| IBIS file stm32u595_599_5a5_5a9_tfbga216_dsi_smps.ibs
[IBIS ver] 4.2
[File name] stm32u595_599_5a5_5a9_tfbga216_dsi_smps.ibs
[File Rev] rev2.0
[Date]  11-09-2023
[Source] Data Created at STMicroelectronics
[Notes]  File originated from ELDO simulations.
[Disclaimer]  This information is for modeling purpose only and is
   not guaranteed. The information is subject to change without
   notice.
[Copyright] Copyright 2023 STMicroelectronics Inc.
|   Component stm32u595_599_5a5_5a9_tfbga216_dsi_smps
[Component] stm32u595_599_5a5_5a9_tfbga216_dsi_smps
[Manufacturer] STMicroelectronics
[Package]
| variable   typ   min   max
R_pkg  0  NA  NA
L_pkg  0  NA  NA
C_pkg  0  NA  NA
[Pin]   signal_name   model_name
A1  VSS  gnd
A2  PE0  io8_100m_hslv_ft
A3  PB7  io8_spi_hslv_ft
A4  PB6  io8_100m_i2c_ft
A5  PG15  io8_100m_hslv_ft
A6  PG12  io8_100m_hslv_ft
A7  PG9  io8_100m_hslv_ft
A8  PD4  io8_100m_hslv_ft
A9  PD3  io8_166m_hslv_ft
A10  PC10  io8_100m_ft
A11  PA15  nc
A12  PA14  io8_100m_ft
A13  PA8  io8_166m_hslv_ft
A14  PC8  io8_100m_ft
A15  VSS  gnd
B1  PC14-OSC32_IN  nc
B2  PE4  io8_100m_hslv_tamp_ft
B3  PE1  io8_100m_hslv_ft
B4  PH3-BOOT0  nc
B5  PB5  io8_166m_hslv_ft
B6  PG13  io8_100m_hslv_ft
B7  PG10  io8_100m_hslv_ft
B8  PD5  io8_100m_hslv_ft
B9  PD2  io8_100m_ft
B10  PC11  io8_100m_hslv_ft
B11  PH7  io8_spi_hslv_ft
B12  PH5  io8_100m_i2c_ft
B13  PA12  io8_100m_ft
B14  PA11  io8_100m_ft
B15  PC7  io8_100m_ft
C1  PC15-OSC32_OUT  nc
C2  VBAT  power
C3  PE3  io8_100m_hslv_tamp_ft
C4  PI5  io8_100m_hslv_ft
C5  PB9  io8_100m_i2c_ft
C6  PB8  io8_100m_i2c_ft
C7  PG11  io8_100m_hslv_ft
C8  PD6  io8_166m_hslv_ft
C9  PD1  io8_100m_hslv_ft
C10  PC12  io8_166m_hslv_ft
C11  PH6  io8_166m_hslv_ft
C12  PH4  io8_100m_hslv_ft
C13  PA13  io8_100m_ft
C14  PC9  io8_100m_ft
C15  PC6  io8_100m_ft
D1  PJ3  io8_100m_ft
D2  PJ2  io8_100m_ft
D3  PE5  io8_100m_hslv_tamp_ft
D4  PI7  io8_spi_ft
D5  PI6  io8_spi_ft
D6  PB4  io8_100m_i2c_ft
D7  PG14  io8_100m_hslv_ft
D8  PD7  io8_100m_hslv_ft
D9  PD0  io8_100m_hslv_ft
D10  PH8  io8_100m_hslv_ft
D11  PH2  io8_100m_hslv_ft
D12  PA10  io8_100m_usb_id
D13  PG7  io8_100m_hslv_ft
D14  PG6  io8_100m_hslv_ft
D15  PG3  io8_100m_hslv_ft
E1  PJ7  io8_100m_ft
E2  PJ6  io8_100m_ft
E3  PJ4  io8_100m_ft
E4  PE6  io8_100m_hslv_tamp_ft
E5  PE2  io8_100m_hslv_ft
E6  VDD11  nc
E7  PB3  io8_100m_i2c_ft
E8  VDDIO2  power
E9  VDDUSB  power
E10  VSS  gnd
E11  VDD11  nc
E12  PA9  io8_100m_usb_vbus_ft
E13  PG8  io8_100m_i2c_ft
E14  PG5  io8_100m_hslv_ft
E15  PJ0  io8_spi_ft
F1  PJ10  io8_100m_ft
F2  PJ8  io8_100m_ft
F3  PJ5  io8_100m_ft
F4  PC13  io8_100m_ft
F5  VDD  power
F6  VSS  gnd
F7  VSS  gnd
F8  VDD  power
F9  VSS  gnd
F10  VSS  gnd
F11  VDD11USB  nc
F12  PG4  io8_100m_hslv_ft
F13  PI15  io8_spi_ft
F14  PI14  io8_spi_ft
F15  PI13  io8_spi_ft
G1  DSI_D0P  nc
G2  DSI_D0N  nc
G3  PJ11  io8_100m_ft
G4  PJ1  io8_100m_ft
G5  VDDDSI  nc
G6  VSSDSI  nc
G10  VSS  gnd
G11  VDDIO2  power
G12  PG2  io8_100m_hslv_ft
G13  PI12  io8_spi_ft
G14  PI11  io8_spi_ft
G15  PI10  io8_spi_ft
H1  DSI_CKP  nc
H2  VSSDSI  nc
H3  PF0  io8_100m_hslv_ft
H4  PJ9  io8_100m_ft
H5  VDD11DSI  nc
H6  VSSDSI  nc
H10  VSS  gnd
H11  VDD  power
H12  PI9  io8_spi_ft
H13  PI8  io8_spi_ft
H14  PI4  io8_spi_ft
H15  VSS  gnd
J1  DSI_CKN  nc
J2  VSSDSI  nc
J3  PF2  io8_100m_hslv_ft
J4  PF1  io8_100m_hslv_ft
J5  VDD  power
J6  VSS  gnd
J10  VSS  gnd
J11  VDD_HSPI  power
J12  PI1  io8_spi_ft
J13  PI2  io8_spi_ft
J14  PI3  io8_spi_ft
J15  VSS  gnd
K1  DSI_D1N  nc
K2  DSI_D1P  nc
K3  PF4  io8_spi_ft
K4  PF3  io8_100m_hslv_ft
K5  VREFM  nc
K6  VSSA  nc
K7  VSS  gnd
K8  VSS  gnd
K9  VSS  gnd
K10  VSS  gnd
K11  VDD  power
K12  PD15  io8_100m_hslv_ft
K13  PH14  io8_spi_ft
K14  PH15  io8_spi_ft
K15  PI0  io8_spi_ft
L1  PF10  io8_166m_hslv_ft
L2  PF5  io8_spi_ft
L3  PF7  io8_100m_hslv_ft
L4  PF9  io8_100m_hslv_ft
L5  VREFP  nc
L6  VDDA  nc
L7  VDD  power
L8  VDD  power
L9  VDD  power
L10  VSS  gnd
L11  VDD power
L12  PD11  io8_100m_hslv_ft
L13  PH10  io8_spi_ft
L14  PH11  io8_spi_ft
L15  PH13  io8_spi_ft
M1  PC1  io8_spi_hslv_ft
M2  PF6  io8_100m_hslv_ft
M3  PF8  io8_100m_hslv_ft
M4  PA2  io8_100m_hslv_ft
M5  PA4  io8_100m_hslv_ft
M6  PB1  io8_100m_hslv_ft
M7  PF13  io8_100m_hslv_ft
M8  PE8  io8_100m_hslv_ft
M9  PE13  io8_100m_hslv_ft
M10  PB11  io8_100m_hslv_ft
M11  PB12  io8_166m_hslv_ft
M12  PB13  io8_100m_i2c_ft
M13  PD12  io8_100m_hslv_ft
M14  PH9  io8_spi_ft
M15  PH12  io8_spi_ft
N1  PH0-OSC_IN  nc
N2  PH1-OSC_OUT  nc
N3  PC3  io8_100m_hslv_ft
N4  PA0  io8_100m_hslv_tamp_ft
N5  OPAMP2_VINM  nc
N6  PB0  io8_100m_hslv_ft
N7  PF12  io8_100m_hslv_ft
N8  PG1  io8_100m_hslv_ft
N9  PE7  io8_100m_hslv_ft
N10  PE15  io8_100m_hslv_ft
N11  PE12  io8_100m_hslv_ft
N12  PB10  io8_spi_hslv_ft
N13  PD8  io8_100m_hslv_ft
N14  PD13  io8_100m_hslv_ft
N15  PD14  io8_100m_hslv_ft
P1  PC2  io8_100m_hslv_ft
P2  PC0  io8_100m_hslv_ft
P3  PA1  io8_100m_hslv_tamp_ft
P4  PA3  io8_166m_hslv_ft
P5  PA6  io8_100m_hslv_ft
P6  PC5  io8_100m_tamp_ft
P7  PF11  io8_166m_hslv_ft
P8  PF15  io8_100m_hslv_ft
P9  PE9  io8_166m_hslv_ft
P10  PE10  io8_166m_hslv_ft
P11  PE11  io8_100m_hslv_ft
P12  VSSSMPS  nc
P13  PB14  io8_100m_i2c_ft
P14  PD10  io8_100m_hslv_ft
P15  PD9  io8_100m_hslv_ft
R1  VSS  gnd
R2  NRST  nc
R3  OPAMP1_VINM  nc
R4  PA5  io8_100m_ft
R5  PA7  io8_100m_hslv_ft
R6  PC4  io8_100m_hslv_ft
R7  PB2  io8_100m_hslv_tamp_ft
R8  PF14  io8_100m_hslv_ft
R9  PG0  io8_100m_hslv_ft
R10  PE14  io8_100m_hslv_ft
R11  VLXSMPS  nc
R12  VDDSMPS  nc
R13  VDD11  nc
R14  PB15  nc
R15  VSS  gnd
[Package Model]   481-tfbga-13x13-216-220909
[Pin Mapping]   pulldown_ref   pullup_ref   | Comment
A1  gndio  nc
A2  gndio  vddiom
A3  gndio  vddiom
A4  gndio  vddiom
A5  gndio  vddiom  | Depending on IO usage
| A5  gndio  vddio2  | Depending on IO usage
A6  gndio  vddiom  | Depending on IO usage
| A6  gndio  vddio2  | Depending on IO usage
A7  gndio  vddiom  | Depending on IO usage
| A7  gndio  vddio2  | Depending on IO usage
A8  gndio  vddiom
A9  gndio  vddiom
A10  gndio  vddiom
A11  nc  nc
A12  gndio  vddiom
A13  gndio  vddiom
A14  gndio  vddiom
A15  gndio  nc
B1  nc  nc
B2  gndio  vddiom
B3  gndio  vddiom
B4  nc  nc
B5  gndio  vddiom
B6  gndio  vddiom  | Depending on IO usage
| B6  gndio  vddio2  | Depending on IO usage
B7  gndio  vddiom  | Depending on IO usage
| B7  gndio  vddio2  | Depending on IO usage
B8  gndio  vddiom
B9  gndio  vddiom
B10  gndio  vddiom
B11  gndio  vddiom
B12  gndio  vddiom
B13  gndio  vddiom  | Depending on IO usage
| B13  gndio  vddusb  | Depending on IO usage
B14  gndio  vddiom  | Depending on IO usage
| B14  gndio  vddusb  | Depending on IO usage
B15  gndio  vddiom
C1  nc  nc
C2  nc  vsw
C3  gndio  vddiom
C4  gndio  vddiom
C5  gndio  vddiom
C6  gndio  vddiom
C7  gndio  vddiom  | Depending on IO usage
| C7  gndio  vddio2  | Depending on IO usage
C8  gndio  vddiom
C9  gndio  vddiom
C10  gndio  vddiom
C11  gndio  vddiom
C12  gndio  vddiom
C13  gndio  vddiom  | Depending on IO usage
| C13  gndio  vddusb  | Depending on IO usage
C14  gndio  vddiom
C15  gndio  vddiom
D1  gndio  vddiom
D2  gndio  vddiom
D3  gndio  vddiom
D4  gndio  vddiom
D5  gndio  vddiom
D6  gndio  vddiom
D7  gndio  vddiom  | Depending on IO usage
| D7  gndio  vddio2  | Depending on IO usage
D8  gndio  vddiom
D9  gndio  vddiom
D10  gndio  vddiom
D11  gndio  vddiom
D12  gndio  vddiom  | Depending on IO usage
| D12  gndio  vddusb  | Depending on IO usage
D13  gndio  vddiom  | Depending on IO usage
| D13  gndio  vddio2  | Depending on IO usage
D14  gndio  vddiom  | Depending on IO usage
| D14  gndio  vddio2  | Depending on IO usage
D15  gndio  vddiom  | Depending on IO usage
| D15  gndio  vddio2  | Depending on IO usage
E1  gndio  vddiom
E2  gndio  vddiom
E3  gndio  vddiom
E4  gndio  vddiom
E5  gndio  vddiom
E6  nc  nc
E7  gndio  vddiom
E8  nc  vddio2
E9  nc  vddusb
E10  gndio  nc
E11  nc  nc
E12  gndio  vddiom  | Depending on IO usage
| E12  gndio  vddusb  | Depending on IO usage
E13  gndio  vddiom  | Depending on IO usage
| E13  gndio  vddio2  | Depending on IO usage
E14  gndio  vddiom  | Depending on IO usage
| E14  gndio  vddio2  | Depending on IO usage
E15  gndio  vddiom
F1  gndio  vddiom
F2  gndio  vddiom
F3  gndio  vddiom
F4  gndio  vddiom  | Depending on IO usage
| F4  gndio  vsw  | Depending on IO usage
F5  nc  vddiom
F6  gndio  nc
F7  gndio  nc
F8  nc  vddiom
F9  gndio  nc
F10  gndio  nc
F11  nc  nc
F12  gndio  vddiom  | Depending on IO usage
| F12  gndio  vddio2  | Depending on IO usage
F13  gndio  vddiom
F14  gndio  vddiom
F15  gndio  vddiom
G1  nc  nc
G2  nc  nc
G3  gndio  vddiom
G4  gndio  vddiom
G5  nc  nc
G6  nc  nc
G10  gndio  nc
G11  nc  vddio2
G12  gndio  vddiom  | Depending on IO usage
| G12  gndio  vddio2  | Depending on IO usage
G13  gndio  vddiom
G14  gndio  vddiom
G15  gndio  vddiom
H1  nc  nc
H2  nc  nc
H3  gndio  vddiom
H4  gndio  vddiom
H5  nc  nc
H6  nc  nc
H10  gndio  nc
H11  nc  vddhspi
H12  gndio  vddiom
H13  gndio  vddiom
H14  gndio  vddiom
H15  gndio  nc
J1  nc  nc
J2  nc  nc
J3  gndio  vddiom
J4  gndio  vddiom
J5  nc  vddiom
J6  gndio  nc
J10  gndio  nc
J11  nc  vddhspi
J12  gndio  vddiom
J13  gndio  vddiom
J14  gndio  vddiom
J15  gndio  nc
K1  nc  nc
K2  nc  nc
K3  gndio  vddiom
K4  gndio  vddiom
K5  nc  nc
K6  nc  nc
K7  gndio  nc
K8  gndio  nc
K9  gndio  nc
K10  gndio  nc
K11  nc  vddhspi
K12  gndio  vddiom
K13  gndio  vddiom
K14  gndio  vddiom
K15  gndio  vddiom
L1  gndio  vddiom
L2  gndio  vddiom
L3  gndio  vddiom
L4  gndio  vddiom
L5  nc  nc
L6  nc  nc
L7  nc  vddiom
L8  nc  vddiom
L9  nc  vddiom
L10  gndio  nc
L11  nc  vddhspi
L12  gndio  vddiom
L13  gndio  vddiom
L14  gndio  vddiom
L15  gndio  vddiom
M1  gndio  vddiom
M2  gndio  vddiom
M3  gndio  vddiom
M4  gndio  vddiom
M5  gndio  vddiom
M6  gndio  vddiom
M7  gndio  vddiom
M8  gndio  vddiom
M9  gndio  vddiom
M10  gndio  vddiom
M11  gndio  vddiom
M12  gndio  vddiom
M13  gndio  vddiom
M14  gndio  vddiom
M15  gndio  vddiom
N1  nc  nc
N2  nc  nc
N3  gndio  vddiom
N4  gndio  vddiom
N5  nc  nc
N6  gndio  vddiom
N7  gndio  vddiom
N8  gndio  vddiom
N9  gndio  vddiom
N10  gndio  vddiom
N11  gndio  vddiom
N12  gndio  vddiom
N13  gndio  vddiom
N14  gndio  vddiom
N15  gndio  vddiom
P1  gndio  vddiom
P2  gndio  vddiom
P3  gndio  vddiom
P4  gndio  vddiom
P5  gndio  vddiom
P6  gndio  vddiom
P7  gndio  vddiom
P8  gndio  vddiom
P9  gndio  vddiom
P10  gndio  vddiom
P11  gndio  vddiom
P12  nc  nc
P13  gndio  vddiom
P14  gndio  vddiom
P15  gndio  vddiom
R1  gndio  nc
R2  nc  nc
R3  nc  nc
R4  gndio  vddiom
R5  gndio  vddiom
R6  gndio  vddiom
R7  gndio  vddiom
R8  gndio  vddiom
R9  gndio  vddiom
R10  gndio  vddiom
R11  nc  nc
R12  nc  nc
R13  nc  nc
R14  nc  nc
R15  gndio  nc
[Model Selector] io8_100m_ft
io8_100m_ft_hs_1v2  "IO8_FT 100MHz high speed @ 1.2V"
io8_100m_ft_fs_1v2  "IO8_FT 100MHz fast speed @ 1.2V"
io8_100m_ft_fs_pd_1v2  "IO8_FT 100MHz fast speed @ 1.2V pulldown"
io8_100m_ft_ms_1v2  "IO8_FT 100MHz med speed @ 1.2V"
io8_100m_ft_ms_pd_1v2  "IO8_FT 100MHz med speed @ 1.2V pulldown"
io8_100m_ft_ls_1v2  "IO8_FT 100MHz low speed @ 1.2V"
io8_100m_ft_ls_pd_1v2  "IO8_FT 100MHz low speed @ 1.2V pulldown"
io8_100m_ft_hs_1v8  "IO8_FT 100MHz high speed @ 1.8V"
io8_100m_ft_hs_pd_1v8  "IO8_FT 100MHz high speed @ 1.8V pulldown"
io8_100m_ft_fs_1v8  "IO8_FT 100MHz fast speed @ 1.8V"
io8_100m_ft_fs_pd_1v8  "IO8_FT 100MHz fast speed @ 1.8V pulldown"
io8_100m_ft_ms_1v8  "IO8_FT 100MHz med speed @ 1.8V"
io8_100m_ft_ms_pd_1v8  "IO8_FT 100MHz med speed @ 1.8V pulldown"
io8_100m_ft_ls_1v8  "IO8_FT 100MHz low speed @ 1.8V"
io8_100m_ft_ls_pd_1v8  "IO8_FT 100MHz low speed @ 1.8V pulldown"
io8_100m_ft_hs_3v3  "IO8_FT 100MHz high speed @ 3.3V"
io8_100m_ft_hs_pd_3v3  "IO8_FT 100MHz high speed @ 3.3V pulldown"
io8_100m_ft_fs_3v3  "IO8_FT 100MHz fast speed @ 3.3V"
io8_100m_ft_fs_pd_3v3  "IO8_FT 100MHz fast speed @ 3.3V pulldown"
io8_100m_ft_ms_3v3  "IO8_FT 100MHz med speed @ 3.3V"
io8_100m_ft_ms_pd_3v3  "IO8_FT 100MHz med speed @ 3.3V pulldown"
io8_100m_ft_ls_3v3  "IO8_FT 100MHz low speed @ 3.3V"
io8_100m_ft_ls_pd_3v3  "IO8_FT 100MHz low speed @ 3.3V pulldown"
[Model Selector] io8_100m_hslv_ft
io8_100m_ft_hs_1v2  "IO8_FT 100MHz high speed @ 1.2V"
io8_100m_ft_hs_pu_1v2  "IO8_FT 100MHz high speed @ 1.2V pullup"
io8_100m_ft_hs_pd_1v2  "IO8_FT 100MHz high speed @ 1.2V pulldown"
io8_100m_ft_fs_1v2  "IO8_FT 100MHz fast speed @ 1.2V"
io8_100m_ft_fs_pu_1v2  "IO8_FT 100MHz fast speed @ 1.2V pullup"
io8_100m_ft_fs_pd_1v2  "IO8_FT 100MHz fast speed @ 1.2V pulldown"
io8_100m_ft_ms_1v2  "IO8_FT 100MHz med speed @ 1.2V"
io8_100m_ft_ms_pu_1v2  "IO8_FT 100MHz med speed @ 1.2V pullup"
io8_100m_ft_ms_pd_1v2  "IO8_FT 100MHz med speed @ 1.2V pulldown"
io8_100m_ft_ls_1v2  "IO8_FT 100MHz low speed @ 1.2V"
io8_100m_ft_ls_pu_1v2  "IO8_FT 100MHz low speed @ 1.2V pullup"
io8_100m_ft_ls_pd_1v2  "IO8_FT 100MHz low speed @ 1.2V pulldown"
io8_100m_ft_hs_1v8  "IO8_FT 100MHz high speed @ 1.8V"
io8_100m_ft_hs_pu_1v8  "IO8_FT 100MHz high speed @ 1.8V pullup"
io8_100m_ft_hs_pd_1v8  "IO8_FT 100MHz high speed @ 1.8V pulldown"
io8_100m_ft_fs_1v8  "IO8_FT 100MHz fast speed @ 1.8V"
io8_100m_ft_fs_pu_1v8  "IO8_FT 100MHz fast speed @ 1.8V pullup"
io8_100m_ft_fs_pd_1v8  "IO8_FT 100MHz fast speed @ 1.8V pulldown"
io8_100m_ft_ms_1v8  "IO8_FT 100MHz med speed @ 1.8V"
io8_100m_ft_ms_pu_1v8  "IO8_FT 100MHz med speed @ 1.8V pullup"
io8_100m_ft_ms_pd_1v8  "IO8_FT 100MHz med speed @ 1.8V pulldown"
io8_100m_ft_ls_1v8  "IO8_FT 100MHz low speed @ 1.8V"
io8_100m_ft_ls_pu_1v8  "IO8_FT 100MHz low speed @ 1.8V pullup"
io8_100m_ft_ls_pd_1v8  "IO8_FT 100MHz low speed @ 1.8V pulldown"
io8_100m_ft_hs_3v3  "IO8_FT 100MHz high speed @ 3.3V"
io8_100m_ft_hs_pu_3v3  "IO8_FT 100MHz high speed @ 3.3V pullup"
io8_100m_ft_hs_pd_3v3  "IO8_FT 100MHz high speed @ 3.3V pulldown"
io8_100m_ft_fs_3v3  "IO8_FT 100MHz fast speed @ 3.3V"
io8_100m_ft_fs_pu_3v3  "IO8_FT 100MHz fast speed @ 3.3V pullup"
io8_100m_ft_fs_pd_3v3  "IO8_FT 100MHz fast speed @ 3.3V pulldown"
io8_100m_ft_ms_3v3  "IO8_FT 100MHz med speed @ 3.3V"
io8_100m_ft_ms_pu_3v3  "IO8_FT 100MHz med speed @ 3.3V pullup"
io8_100m_ft_ms_pd_3v3  "IO8_FT 100MHz med speed @ 3.3V pulldown"
io8_100m_ft_ls_3v3  "IO8_FT 100MHz low speed @ 3.3V"
io8_100m_ft_ls_pu_3v3  "IO8_FT 100MHz low speed @ 3.3V pullup"
io8_100m_ft_ls_pd_3v3  "IO8_FT 100MHz low speed @ 3.3V pulldown"
io8_100m_hslv_ft_hs_1v2  "IO8_FT 100MHz HSLV high speed @ 1.2V"
io8_100m_hslv_ft_hs_pu_1v2  "IO8_FT 100MHz HSLV high speed @ 1.2V pullup"
io8_100m_hslv_ft_hs_pd_1v2  "IO8_FT 100MHz HSLV high speed @ 1.2V pulldown"
io8_100m_hslv_ft_fs_1v2  "IO8_FT 100MHz HSLV fast speed @ 1.2V"
io8_100m_hslv_ft_fs_pu_1v2  "IO8_FT 100MHz HSLV fast speed @ 1.2V pullup"
io8_100m_hslv_ft_fs_pd_1v2  "IO8_FT 100MHz HSLV fast speed @ 1.2V pulldown"
io8_100m_hslv_ft_ms_1v2  "IO8_FT 100MHz HSLV med speed @ 1.2V"
io8_100m_hslv_ft_ms_pu_1v2  "IO8_FT 100MHz HSLV med speed @ 1.2V pullup"
io8_100m_hslv_ft_ms_pd_1v2  "IO8_FT 100MHz HSLV med speed @ 1.2V pulldown"
io8_100m_hslv_ft_ls_1v2  "IO8_FT 100MHz HSLV low speed @ 1.2V"
io8_100m_hslv_ft_ls_pu_1v2  "IO8_FT 100MHz HSLV low speed @ 1.2V pullup"
io8_100m_hslv_ft_ls_pd_1v2  "IO8_FT 100MHz HSLV low speed @ 1.2V pulldown"
io8_100m_hslv_ft_hs_1v8  "IO8_FT 100MHz HSLV high speed @ 1.8V"
io8_100m_hslv_ft_hs_pu_1v8  "IO8_FT 100MHz HSLV high speed @ 1.8V pullup"
io8_100m_hslv_ft_hs_pd_1v8  "IO8_FT 100MHz HSLV high speed @ 1.8V pulldown"
io8_100m_hslv_ft_fs_1v8  "IO8_FT 100MHz HSLV fast speed @ 1.8V"
io8_100m_hslv_ft_fs_pu_1v8  "IO8_FT 100MHz HSLV fast speed @ 1.8V pullup"
io8_100m_hslv_ft_fs_pd_1v8  "IO8_FT 100MHz HSLV fast speed @ 1.8V pulldown"
io8_100m_hslv_ft_ms_1v8  "IO8_FT 100MHz HSLV med speed @ 1.8V"
io8_100m_hslv_ft_ms_pu_1v8  "IO8_FT 100MHz HSLV med speed @ 1.8V pullup"
io8_100m_hslv_ft_ms_pd_1v8  "IO8_FT 100MHz HSLV med speed @ 1.8V pulldown"
io8_100m_hslv_ft_ls_1v8  "IO8_FT 100MHz HSLV low speed @ 1.8V"
io8_100m_hslv_ft_ls_pu_1v8  "IO8_FT 100MHz HSLV low speed @ 1.8V pullup"
io8_100m_hslv_ft_ls_pd_1v8  "IO8_FT 100MHz HSLV low speed @ 1.8V pulldown"
io8_100m_hslv_ft_hs_2v5  "IO8_FT 100MHz HSLV high speed @ 2.5V"
io8_100m_hslv_ft_hs_pu_2v5  "IO8_FT 100MHz HSLV high speed @ 2.5V pullup"
io8_100m_hslv_ft_hs_pd_2v5  "IO8_FT 100MHz HSLV high speed @ 2.5V pulldown"
io8_100m_hslv_ft_fs_2v5  "IO8_FT 100MHz HSLV fast speed @ 2.5V"
io8_100m_hslv_ft_fs_pu_2v5  "IO8_FT 100MHz HSLV fast speed @ 2.5V pullup"
io8_100m_hslv_ft_fs_pd_2v5  "IO8_FT 100MHz HSLV fast speed @ 2.5V pulldown"
io8_100m_hslv_ft_ms_2v5  "IO8_FT 100MHz HSLV med speed @ 2.5V"
io8_100m_hslv_ft_ms_pu_2v5  "IO8_FT 100MHz HSLV med speed @ 2.5V pullup"
io8_100m_hslv_ft_ms_pd_2v5  "IO8_FT 100MHz HSLV med speed @ 2.5V pulldown"
io8_100m_hslv_ft_ls_2v5  "IO8_FT 100MHz HSLV low speed @ 2.5V"
io8_100m_hslv_ft_ls_pu_2v5  "IO8_FT 100MHz HSLV low speed @ 2.5V pullup"
io8_100m_hslv_ft_ls_pd_2v5  "IO8_FT 100MHz HSLV low speed @ 2.5V pulldown"
[Model Selector] io8_100m_hslv_tamp_ft
io8_100m_ft_hs_1v2  "IO8_FT 100MHz high speed @ 1.2V"
io8_100m_ft_hs_pu_1v2  "IO8_FT 100MHz high speed @ 1.2V pullup"
io8_100m_ft_hs_pd_1v2  "IO8_FT 100MHz high speed @ 1.2V pulldown"
io8_100m_ft_fs_1v2  "IO8_FT 100MHz fast speed @ 1.2V"
io8_100m_ft_fs_pu_1v2  "IO8_FT 100MHz fast speed @ 1.2V pullup"
io8_100m_ft_fs_pd_1v2  "IO8_FT 100MHz fast speed @ 1.2V pulldown"
io8_100m_ft_ms_1v2  "IO8_FT 100MHz med speed @ 1.2V"
io8_100m_ft_ms_pu_1v2  "IO8_FT 100MHz med speed @ 1.2V pullup"
io8_100m_ft_ms_pd_1v2  "IO8_FT 100MHz med speed @ 1.2V pulldown"
io8_100m_ft_ls_1v2  "IO8_FT 100MHz low speed @ 1.2V"
io8_100m_ft_ls_pu_1v2  "IO8_FT 100MHz low speed @ 1.2V pullup"
io8_100m_ft_ls_pd_1v2  "IO8_FT 100MHz low speed @ 1.2V pulldown"
io8_100m_ft_hs_1v8  "IO8_FT 100MHz high speed @ 1.8V"
io8_100m_ft_hs_pu_1v8  "IO8_FT 100MHz high speed @ 1.8V pullup"
io8_100m_ft_hs_pd_1v8  "IO8_FT 100MHz high speed @ 1.8V pulldown"
io8_100m_ft_fs_1v8  "IO8_FT 100MHz fast speed @ 1.8V"
io8_100m_ft_fs_pu_1v8  "IO8_FT 100MHz fast speed @ 1.8V pullup"
io8_100m_ft_fs_pd_1v8  "IO8_FT 100MHz fast speed @ 1.8V pulldown"
io8_100m_ft_ms_1v8  "IO8_FT 100MHz med speed @ 1.8V"
io8_100m_ft_ms_pu_1v8  "IO8_FT 100MHz med speed @ 1.8V pullup"
io8_100m_ft_ms_pd_1v8  "IO8_FT 100MHz med speed @ 1.8V pulldown"
io8_100m_ft_ls_1v8  "IO8_FT 100MHz low speed @ 1.8V"
io8_100m_ft_ls_pu_1v8  "IO8_FT 100MHz low speed @ 1.8V pullup"
io8_100m_ft_ls_pd_1v8  "IO8_FT 100MHz low speed @ 1.8V pulldown"
io8_100m_ft_hs_3v3  "IO8_FT 100MHz high speed @ 3.3V"
io8_100m_ft_hs_pu_3v3  "IO8_FT 100MHz high speed @ 3.3V pullup"
io8_100m_ft_hs_pd_3v3  "IO8_FT 100MHz high speed @ 3.3V pulldown"
io8_100m_ft_fs_3v3  "IO8_FT 100MHz fast speed @ 3.3V"
io8_100m_ft_fs_pu_3v3  "IO8_FT 100MHz fast speed @ 3.3V pullup"
io8_100m_ft_fs_pd_3v3  "IO8_FT 100MHz fast speed @ 3.3V pulldown"
io8_100m_ft_ms_3v3  "IO8_FT 100MHz med speed @ 3.3V"
io8_100m_ft_ms_pu_3v3  "IO8_FT 100MHz med speed @ 3.3V pullup"
io8_100m_ft_ms_pd_3v3  "IO8_FT 100MHz med speed @ 3.3V pulldown"
io8_100m_ft_ls_3v3  "IO8_FT 100MHz low speed @ 3.3V"
io8_100m_ft_ls_pu_3v3  "IO8_FT 100MHz low speed @ 3.3V pullup"
io8_100m_ft_ls_pd_3v3  "IO8_FT 100MHz low speed @ 3.3V pulldown"
io8_100m_hslv_ft_hs_1v2  "IO8_FT 100MHz HSLV high speed @ 1.2V"
io8_100m_hslv_ft_hs_pu_1v2  "IO8_FT 100MHz HSLV high speed @ 1.2V pullup"
io8_100m_hslv_ft_hs_pd_1v2  "IO8_FT 100MHz HSLV high speed @ 1.2V pulldown"
io8_100m_hslv_ft_fs_1v2  "IO8_FT 100MHz HSLV fast speed @ 1.2V"
io8_100m_hslv_ft_fs_pu_1v2  "IO8_FT 100MHz HSLV fast speed @ 1.2V pullup"
io8_100m_hslv_ft_fs_pd_1v2  "IO8_FT 100MHz HSLV fast speed @ 1.2V pulldown"
io8_100m_hslv_ft_ms_1v2  "IO8_FT 100MHz HSLV med speed @ 1.2V"
io8_100m_hslv_ft_ms_pu_1v2  "IO8_FT 100MHz HSLV med speed @ 1.2V pullup"
io8_100m_hslv_ft_ms_pd_1v2  "IO8_FT 100MHz HSLV med speed @ 1.2V pulldown"
io8_100m_hslv_ft_ls_1v2  "IO8_FT 100MHz HSLV low speed @ 1.2V"
io8_100m_hslv_ft_ls_pu_1v2  "IO8_FT 100MHz HSLV low speed @ 1.2V pullup"
io8_100m_hslv_ft_ls_pd_1v2  "IO8_FT 100MHz HSLV low speed @ 1.2V pulldown"
io8_100m_hslv_ft_hs_1v8  "IO8_FT 100MHz HSLV high speed @ 1.8V"
io8_100m_hslv_ft_hs_pu_1v8  "IO8_FT 100MHz HSLV high speed @ 1.8V pullup"
io8_100m_hslv_ft_hs_pd_1v8  "IO8_FT 100MHz HSLV high speed @ 1.8V pulldown"
io8_100m_hslv_ft_fs_1v8  "IO8_FT 100MHz HSLV fast speed @ 1.8V"
io8_100m_hslv_ft_fs_pu_1v8  "IO8_FT 100MHz HSLV fast speed @ 1.8V pullup"
io8_100m_hslv_ft_fs_pd_1v8  "IO8_FT 100MHz HSLV fast speed @ 1.8V pulldown"
io8_100m_hslv_ft_ms_1v8  "IO8_FT 100MHz HSLV med speed @ 1.8V"
io8_100m_hslv_ft_ms_pu_1v8  "IO8_FT 100MHz HSLV med speed @ 1.8V pullup"
io8_100m_hslv_ft_ms_pd_1v8  "IO8_FT 100MHz HSLV med speed @ 1.8V pulldown"
io8_100m_hslv_ft_ls_1v8  "IO8_FT 100MHz HSLV low speed @ 1.8V"
io8_100m_hslv_ft_ls_pu_1v8  "IO8_FT 100MHz HSLV low speed @ 1.8V pullup"
io8_100m_hslv_ft_ls_pd_1v8  "IO8_FT 100MHz HSLV low speed @ 1.8V pulldown"
io8_100m_hslv_ft_hs_2v5  "IO8_FT 100MHz HSLV high speed @ 2.5V"
io8_100m_hslv_ft_hs_pu_2v5  "IO8_FT 100MHz HSLV high speed @ 2.5V pullup"
io8_100m_hslv_ft_hs_pd_2v5  "IO8_FT 100MHz HSLV high speed @ 2.5V pulldown"
io8_100m_hslv_ft_fs_2v5  "IO8_FT 100MHz HSLV fast speed @ 2.5V"
io8_100m_hslv_ft_fs_pu_2v5  "IO8_FT 100MHz HSLV fast speed @ 2.5V pullup"
io8_100m_hslv_ft_fs_pd_2v5  "IO8_FT 100MHz HSLV fast speed @ 2.5V pulldown"
io8_100m_hslv_ft_ms_2v5  "IO8_FT 100MHz HSLV med speed @ 2.5V"
io8_100m_hslv_ft_ms_pu_2v5  "IO8_FT 100MHz HSLV med speed @ 2.5V pullup"
io8_100m_hslv_ft_ms_pd_2v5  "IO8_FT 100MHz HSLV med speed @ 2.5V pulldown"
io8_100m_hslv_ft_ls_2v5  "IO8_FT 100MHz HSLV low speed @ 2.5V"
io8_100m_hslv_ft_ls_pu_2v5  "IO8_FT 100MHz HSLV low speed @ 2.5V pullup"
io8_100m_hslv_ft_ls_pd_2v5  "IO8_FT 100MHz HSLV low speed @ 2.5V pulldown"
io8_ft_v33_hs_1v2  "IO8_FT_V33 high speed @ 1.2V"
io8_ft_v33_hs_pu_1v2  "IO8_FT_V33 high speed @ 1.2V pullup"
io8_ft_v33_hs_pd_1v2  "IO8_FT_V33 high speed @ 1.2V pulldown"
io8_ft_v33_fs_1v2  "IO8_FT_V33 fast speed @ 1.2V"
io8_ft_v33_fs_pu_1v2  "IO8_FT_V33 fast speed @ 1.2V pullup"
io8_ft_v33_fs_pd_1v2  "IO8_FT_V33 fast speed @ 1.2V pulldown"
io8_ft_v33_ms_1v2  "IO8_FT_V33 med speed @ 1.2V"
io8_ft_v33_ms_pu_1v2  "IO8_FT_V33 med speed @ 1.2V pullup"
io8_ft_v33_ms_pd_1v2  "IO8_FT_V33 med speed @ 1.2V pulldown"
io8_ft_v33_ls_1v2  "IO8_FT_V33 low speed @ 1.2V"
io8_ft_v33_ls_pu_1v2  "IO8_FT_V33 low speed @ 1.2V pullup"
io8_ft_v33_ls_pd_1v2  "IO8_FT_V33 low speed @ 1.2V pulldown"
io8_ft_v33_hs_1v8  "IO8_FT_V33 high speed @ 1.8V"
io8_ft_v33_hs_pu_1v8  "IO8_FT_V33 high speed @ 1.8V pullup"
io8_ft_v33_hs_pd_1v8  "IO8_FT_V33 high speed @ 1.8V pulldown"
io8_ft_v33_fs_1v8  "IO8_FT_V33 fast speed @ 1.8V"
io8_ft_v33_fs_pu_1v8  "IO8_FT_V33 fast speed @ 1.8V pullup"
io8_ft_v33_fs_pd_1v8  "IO8_FT_V33 fast speed @ 1.8V pulldown"
io8_ft_v33_ms_1v8  "IO8_FT_V33 med speed @ 1.8V"
io8_ft_v33_ms_pu_1v8  "IO8_FT_V33 med speed @ 1.8V pullup"
io8_ft_v33_ms_pd_1v8  "IO8_FT_V33 med speed @ 1.8V pulldown"
io8_ft_v33_ls_1v8  "IO8_FT_V33 low speed @ 1.8V"
io8_ft_v33_ls_pu_1v8  "IO8_FT_V33 low speed @ 1.8V pullup"
io8_ft_v33_ls_pd_1v8  "IO8_FT_V33 low speed @ 1.8V pulldown"
io8_ft_v33_hs_3v3  "IO8_FT_V33 high speed @ 3.3V"
io8_ft_v33_hs_pu_3v3  "IO8_FT_V33 high speed @ 3.3V pullup"
io8_ft_v33_hs_pd_3v3  "IO8_FT_V33 high speed @ 3.3V pulldown"
io8_ft_v33_fs_3v3  "IO8_FT_V33 fast speed @ 3.3V"
io8_ft_v33_fs_pu_3v3  "IO8_FT_V33 fast speed @ 3.3V pullup"
io8_ft_v33_fs_pd_3v3  "IO8_FT_V33 fast speed @ 3.3V pulldown"
io8_ft_v33_ms_3v3  "IO8_FT_V33 med speed @ 3.3V"
io8_ft_v33_ms_pu_3v3  "IO8_FT_V33 med speed @ 3.3V pullup"
io8_ft_v33_ms_pd_3v3  "IO8_FT_V33 med speed @ 3.3V pulldown"
io8_ft_v33_ls_3v3  "IO8_FT_V33 low speed @ 3.3V"
io8_ft_v33_ls_pu_3v3  "IO8_FT_V33 low speed @ 3.3V pullup"
io8_ft_v33_ls_pd_3v3  "IO8_FT_V33 low speed @ 3.3V pulldown"
[Model Selector] io8_100m_i2c_ft
io8_100m_ft_hs_1v2  "IO8_FT 100MHz high speed @ 1.2V"
io8_100m_ft_hs_pu_1v2  "IO8_FT 100MHz high speed @ 1.2V pullup"
io8_100m_ft_hs_pd_1v2  "IO8_FT 100MHz high speed @ 1.2V pulldown"
io8_100m_ft_fs_1v2  "IO8_FT 100MHz fast speed @ 1.2V"
io8_100m_ft_fs_pu_1v2  "IO8_FT 100MHz fast speed @ 1.2V pullup"
io8_100m_ft_fs_pd_1v2  "IO8_FT 100MHz fast speed @ 1.2V pulldown"
io8_100m_ft_ms_1v2  "IO8_FT 100MHz med speed @ 1.2V"
io8_100m_ft_ms_pu_1v2  "IO8_FT 100MHz med speed @ 1.2V pullup"
io8_100m_ft_ms_pd_1v2  "IO8_FT 100MHz med speed @ 1.2V pulldown"
io8_100m_ft_ls_1v2  "IO8_FT 100MHz low speed @ 1.2V"
io8_100m_ft_ls_pu_1v2  "IO8_FT 100MHz low speed @ 1.2V pullup"
io8_100m_ft_ls_pd_1v2  "IO8_FT 100MHz low speed @ 1.2V pulldown"
io8_100m_ft_hs_1v8  "IO8_FT 100MHz high speed @ 1.8V"
io8_100m_ft_hs_pu_1v8  "IO8_FT 100MHz high speed @ 1.8V pullup"
io8_100m_ft_hs_pd_1v8  "IO8_FT 100MHz high speed @ 1.8V pulldown"
io8_100m_ft_fs_1v8  "IO8_FT 100MHz fast speed @ 1.8V"
io8_100m_ft_fs_pu_1v8  "IO8_FT 100MHz fast speed @ 1.8V pullup"
io8_100m_ft_fs_pd_1v8  "IO8_FT 100MHz fast speed @ 1.8V pulldown"
io8_100m_ft_ms_1v8  "IO8_FT 100MHz med speed @ 1.8V"
io8_100m_ft_ms_pu_1v8  "IO8_FT 100MHz med speed @ 1.8V pullup"
io8_100m_ft_ms_pd_1v8  "IO8_FT 100MHz med speed @ 1.8V pulldown"
io8_100m_ft_ls_1v8  "IO8_FT 100MHz low speed @ 1.8V"
io8_100m_ft_ls_pu_1v8  "IO8_FT 100MHz low speed @ 1.8V pullup"
io8_100m_ft_ls_pd_1v8  "IO8_FT 100MHz low speed @ 1.8V pulldown"
io8_100m_ft_hs_3v3  "IO8_FT 100MHz high speed @ 3.3V"
io8_100m_ft_hs_pu_3v3  "IO8_FT 100MHz high speed @ 3.3V pullup"
io8_100m_ft_hs_pd_3v3  "IO8_FT 100MHz high speed @ 3.3V pulldown"
io8_100m_ft_fs_3v3  "IO8_FT 100MHz fast speed @ 3.3V"
io8_100m_ft_fs_pu_3v3  "IO8_FT 100MHz fast speed @ 3.3V pullup"
io8_100m_ft_fs_pd_3v3  "IO8_FT 100MHz fast speed @ 3.3V pulldown"
io8_100m_ft_ms_3v3  "IO8_FT 100MHz med speed @ 3.3V"
io8_100m_ft_ms_pu_3v3  "IO8_FT 100MHz med speed @ 3.3V pullup"
io8_100m_ft_ms_pd_3v3  "IO8_FT 100MHz med speed @ 3.3V pulldown"
io8_100m_ft_ls_3v3  "IO8_FT 100MHz low speed @ 3.3V"
io8_100m_ft_ls_pu_3v3  "IO8_FT 100MHz low speed @ 3.3V pullup"
io8_100m_ft_ls_pd_3v3  "IO8_FT 100MHz low speed @ 3.3V pulldown"
io8_100m_i2c_ft_1v2  "IO8_FT 100MHz I2C @ 1.2V"
io8_100m_i2c_ft_pu_1v2  "IO8_FT 100MHz I2C @ 1.2V pullup"
io8_100m_i2c_ft_pd_1v2  "IO8_FT 100MHz I2C @ 1.2V pulldown"
io8_100m_i2c_ft_1v8  "IO8_FT 100MHz I2C @ 1.8V"
io8_100m_i2c_ft_pu_1v8  "IO8_FT 100MHz I2C @ 1.8V pullup"
io8_100m_i2c_ft_pd_1v8  "IO8_FT 100MHz I2C @ 1,8V pulldown"
io8_100m_i2c_ft_3v3  "IO8_FT 100MHz I2C @ 3.3V"
io8_100m_i2c_ft_pu_3v3  "IO8_FT 100MHz I2C HSLV @ 3.3V pullup"
io8_100m_i2c_ft_pd_3v3  "IO8_FT 100MHz I2C @ 3.3V pulldown"
[Model Selector] io8_100m_tamp_ft
io8_100m_ft_hs_1v2  "IO8_FT 100MHz high speed @ 1.2V"
io8_100m_ft_hs_pu_1v2  "IO8_FT 100MHz high speed @ 1.2V pullup"
io8_100m_ft_hs_pd_1v2  "IO8_FT 100MHz high speed @ 1.2V pulldown"
io8_100m_ft_fs_1v2  "IO8_FT 100MHz fast speed @ 1.2V"
io8_100m_ft_fs_pu_1v2  "IO8_FT 100MHz fast speed @ 1.2V pullup"
io8_100m_ft_fs_pd_1v2  "IO8_FT 100MHz fast speed @ 1.2V pulldown"
io8_100m_ft_ms_1v2  "IO8_FT 100MHz med speed @ 1.2V"
io8_100m_ft_ms_pu_1v2  "IO8_FT 100MHz med speed @ 1.2V pullup"
io8_100m_ft_ms_pd_1v2  "IO8_FT 100MHz med speed @ 1.2V pulldown"
io8_100m_ft_ls_1v2  "IO8_FT 100MHz low speed @ 1.2V"
io8_100m_ft_ls_pu_1v2  "IO8_FT 100MHz low speed @ 1.2V pullup"
io8_100m_ft_ls_pd_1v2  "IO8_FT 100MHz low speed @ 1.2V pulldown"
io8_100m_ft_hs_1v8  "IO8_FT 100MHz high speed @ 1.8V"
io8_100m_ft_hs_pu_1v8  "IO8_FT 100MHz high speed @ 1.8V pullup"
io8_100m_ft_hs_pd_1v8  "IO8_FT 100MHz high speed @ 1.8V pulldown"
io8_100m_ft_fs_1v8  "IO8_FT 100MHz fast speed @ 1.8V"
io8_100m_ft_fs_pu_1v8  "IO8_FT 100MHz fast speed @ 1.8V pullup"
io8_100m_ft_fs_pd_1v8  "IO8_FT 100MHz fast speed @ 1.8V pulldown"
io8_100m_ft_ms_1v8  "IO8_FT 100MHz med speed @ 1.8V"
io8_100m_ft_ms_pu_1v8  "IO8_FT 100MHz med speed @ 1.8V pullup"
io8_100m_ft_ms_pd_1v8  "IO8_FT 100MHz med speed @ 1.8V pulldown"
io8_100m_ft_ls_1v8  "IO8_FT 100MHz low speed @ 1.8V"
io8_100m_ft_ls_pu_1v8  "IO8_FT 100MHz low speed @ 1.8V pullup"
io8_100m_ft_ls_pd_1v8  "IO8_FT 100MHz low speed @ 1.8V pulldown"
io8_100m_ft_hs_3v3  "IO8_FT 100MHz high speed @ 3.3V"
io8_100m_ft_hs_pu_3v3  "IO8_FT 100MHz high speed @ 3.3V pullup"
io8_100m_ft_hs_pd_3v3  "IO8_FT 100MHz high speed @ 3.3V pulldown"
io8_100m_ft_fs_3v3  "IO8_FT 100MHz fast speed @ 3.3V"
io8_100m_ft_fs_pu_3v3  "IO8_FT 100MHz fast speed @ 3.3V pullup"
io8_100m_ft_fs_pd_3v3  "IO8_FT 100MHz fast speed @ 3.3V pulldown"
io8_100m_ft_ms_3v3  "IO8_FT 100MHz med speed @ 3.3V"
io8_100m_ft_ms_pu_3v3  "IO8_FT 100MHz med speed @ 3.3V pullup"
io8_100m_ft_ms_pd_3v3  "IO8_FT 100MHz med speed @ 3.3V pulldown"
io8_100m_ft_ls_3v3  "IO8_FT 100MHz low speed @ 3.3V"
io8_100m_ft_ls_pu_3v3  "IO8_FT 100MHz low speed @ 3.3V pullup"
io8_100m_ft_ls_pd_3v3  "IO8_FT 100MHz low speed @ 3.3V pulldown"
io8_ft_v33_hs_1v2  "IO8_FT_V33 high speed @ 1.2V"
io8_ft_v33_hs_pu_1v2  "IO8_FT_V33 high speed @ 1.2V pullup"
io8_ft_v33_hs_pd_1v2  "IO8_FT_V33 high speed @ 1.2V pulldown"
io8_ft_v33_fs_1v2  "IO8_FT_V33 fast speed @ 1.2V"
io8_ft_v33_fs_pu_1v2  "IO8_FT_V33 fast speed @ 1.2V pullup"
io8_ft_v33_fs_pd_1v2  "IO8_FT_V33 fast speed @ 1.2V pulldown"
io8_ft_v33_ms_1v2  "IO8_FT_V33 med speed @ 1.2V"
io8_ft_v33_ms_pu_1v2  "IO8_FT_V33 med speed @ 1.2V pullup"
io8_ft_v33_ms_pd_1v2  "IO8_FT_V33 med speed @ 1.2V pulldown"
io8_ft_v33_ls_1v2  "IO8_FT_V33 low speed @ 1.2V"
io8_ft_v33_ls_pu_1v2  "IO8_FT_V33 low speed @ 1.2V pullup"
io8_ft_v33_ls_pd_1v2  "IO8_FT_V33 low speed @ 1.2V pulldown"
io8_ft_v33_hs_1v8  "IO8_FT_V33 high speed @ 1.8V"
io8_ft_v33_hs_pu_1v8  "IO8_FT_V33 high speed @ 1.8V pullup"
io8_ft_v33_hs_pd_1v8  "IO8_FT_V33 high speed @ 1.8V pulldown"
io8_ft_v33_fs_1v8  "IO8_FT_V33 fast speed @ 1.8V"
io8_ft_v33_fs_pu_1v8  "IO8_FT_V33 fast speed @ 1.8V pullup"
io8_ft_v33_fs_pd_1v8  "IO8_FT_V33 fast speed @ 1.8V pulldown"
io8_ft_v33_ms_1v8  "IO8_FT_V33 med speed @ 1.8V"
io8_ft_v33_ms_pu_1v8  "IO8_FT_V33 med speed @ 1.8V pullup"
io8_ft_v33_ms_pd_1v8  "IO8_FT_V33 med speed @ 1.8V pulldown"
io8_ft_v33_ls_1v8  "IO8_FT_V33 low speed @ 1.8V"
io8_ft_v33_ls_pu_1v8  "IO8_FT_V33 low speed @ 1.8V pullup"
io8_ft_v33_ls_pd_1v8  "IO8_FT_V33 low speed @ 1.8V pulldown"
io8_ft_v33_hs_3v3  "IO8_FT_V33 high speed @ 3.3V"
io8_ft_v33_hs_pu_3v3  "IO8_FT_V33 high speed @ 3.3V pullup"
io8_ft_v33_hs_pd_3v3  "IO8_FT_V33 high speed @ 3.3V pulldown"
io8_ft_v33_fs_3v3  "IO8_FT_V33 fast speed @ 3.3V"
io8_ft_v33_fs_pu_3v3  "IO8_FT_V33 fast speed @ 3.3V pullup"
io8_ft_v33_fs_pd_3v3  "IO8_FT_V33 fast speed @ 3.3V pulldown"
io8_ft_v33_ms_3v3  "IO8_FT_V33 med speed @ 3.3V"
io8_ft_v33_ms_pu_3v3  "IO8_FT_V33 med speed @ 3.3V pullup"
io8_ft_v33_ms_pd_3v3  "IO8_FT_V33 med speed @ 3.3V pulldown"
io8_ft_v33_ls_3v3  "IO8_FT_V33 low speed @ 3.3V"
io8_ft_v33_ls_pu_3v3  "IO8_FT_V33 low speed @ 3.3V pullup"
io8_ft_v33_ls_pd_3v3  "IO8_FT_V33 low speed @ 3.3V pulldown"
[Model Selector] io8_100m_usb_id
io8_100m_ft_hs_1v2  "IO8_FT 100MHz high speed @ 1.2V"
io8_100m_ft_hs_pu_1v2  "IO8_FT 100MHz high speed @ 1.2V pullup"
io8_100m_ft_hs_pd_1v2  "IO8_FT 100MHz high speed @ 1.2V pulldown"
io8_100m_ft_fs_1v2  "IO8_FT 100MHz fast speed @ 1.2V"
io8_100m_ft_fs_pu_1v2  "IO8_FT 100MHz fast speed @ 1.2V pullup"
io8_100m_ft_fs_pd_1v2  "IO8_FT 100MHz fast speed @ 1.2V pulldown"
io8_100m_ft_ms_1v2  "IO8_FT 100MHz med speed @ 1.2V"
io8_100m_ft_ms_pu_1v2  "IO8_FT 100MHz med speed @ 1.2V pullup"
io8_100m_ft_ms_pd_1v2  "IO8_FT 100MHz med speed @ 1.2V pulldown"
io8_100m_ft_ls_1v2  "IO8_FT 100MHz low speed @ 1.2V"
io8_100m_ft_ls_pu_1v2  "IO8_FT 100MHz low speed @ 1.2V pullup"
io8_100m_ft_ls_pd_1v2  "IO8_FT 100MHz low speed @ 1.2V pulldown"
io8_100m_ft_hs_1v8  "IO8_FT 100MHz high speed @ 1.8V"
io8_100m_ft_hs_pu_1v8  "IO8_FT 100MHz high speed @ 1.8V pullup"
io8_100m_ft_hs_pd_1v8  "IO8_FT 100MHz high speed @ 1.8V pulldown"
io8_100m_ft_fs_1v8  "IO8_FT 100MHz fast speed @ 1.8V"
io8_100m_ft_fs_pu_1v8  "IO8_FT 100MHz fast speed @ 1.8V pullup"
io8_100m_ft_fs_pd_1v8  "IO8_FT 100MHz fast speed @ 1.8V pulldown"
io8_100m_ft_ms_1v8  "IO8_FT 100MHz med speed @ 1.8V"
io8_100m_ft_ms_pu_1v8  "IO8_FT 100MHz med speed @ 1.8V pullup"
io8_100m_ft_ms_pd_1v8  "IO8_FT 100MHz med speed @ 1.8V pulldown"
io8_100m_ft_ls_1v8  "IO8_FT 100MHz low speed @ 1.8V"
io8_100m_ft_ls_pu_1v8  "IO8_FT 100MHz low speed @ 1.8V pullup"
io8_100m_ft_ls_pd_1v8  "IO8_FT 100MHz low speed @ 1.8V pulldown"
io8_100m_ft_hs_3v3  "IO8_FT 100MHz high speed @ 3.3V"
io8_100m_ft_hs_pu_3v3  "IO8_FT 100MHz high speed @ 3.3V pullup"
io8_100m_ft_hs_pd_3v3  "IO8_FT 100MHz high speed @ 3.3V pulldown"
io8_100m_ft_fs_3v3  "IO8_FT 100MHz fast speed @ 3.3V"
io8_100m_ft_fs_pu_3v3  "IO8_FT 100MHz fast speed @ 3.3V pullup"
io8_100m_ft_fs_pd_3v3  "IO8_FT 100MHz fast speed @ 3.3V pulldown"
io8_100m_ft_ms_3v3  "IO8_FT 100MHz med speed @ 3.3V"
io8_100m_ft_ms_pu_3v3  "IO8_FT 100MHz med speed @ 3.3V pullup"
io8_100m_ft_ms_pd_3v3  "IO8_FT 100MHz med speed @ 3.3V pulldown"
io8_100m_ft_ls_3v3  "IO8_FT 100MHz low speed @ 3.3V"
io8_100m_ft_ls_pu_3v3  "IO8_FT 100MHz low speed @ 3.3V pullup"
io8_100m_ft_ls_pd_3v3  "IO8_FT 100MHz low speed @ 3.3V pulldown"
io8usb_id_nopu  "IOUSB ID @ 3.3V"
io8usb_id_pu  "IOUSB ID @ 3.3V pullup"
[Model Selector] io8_100m_usb_vbus_ft
io8_100m_ft_hs_1v2  "IO8_FT 100MHz high speed @ 1.2V"
io8_100m_ft_hs_pu_1v2  "IO8_FT 100MHz high speed @ 1.2V pullup"
io8_100m_ft_hs_pd_1v2  "IO8_FT 100MHz high speed @ 1.2V pulldown"
io8_100m_ft_fs_1v2  "IO8_FT 100MHz fast speed @ 1.2V"
io8_100m_ft_fs_pu_1v2  "IO8_FT 100MHz fast speed @ 1.2V pullup"
io8_100m_ft_fs_pd_1v2  "IO8_FT 100MHz fast speed @ 1.2V pulldown"
io8_100m_ft_ms_1v2  "IO8_FT 100MHz med speed @ 1.2V"
io8_100m_ft_ms_pu_1v2  "IO8_FT 100MHz med speed @ 1.2V pullup"
io8_100m_ft_ms_pd_1v2  "IO8_FT 100MHz med speed @ 1.2V pulldown"
io8_100m_ft_ls_1v2  "IO8_FT 100MHz low speed @ 1.2V"
io8_100m_ft_ls_pu_1v2  "IO8_FT 100MHz low speed @ 1.2V pullup"
io8_100m_ft_ls_pd_1v2  "IO8_FT 100MHz low speed @ 1.2V pulldown"
io8_100m_ft_hs_1v8  "IO8_FT 100MHz high speed @ 1.8V"
io8_100m_ft_hs_pu_1v8  "IO8_FT 100MHz high speed @ 1.8V pullup"
io8_100m_ft_hs_pd_1v8  "IO8_FT 100MHz high speed @ 1.8V pulldown"
io8_100m_ft_fs_1v8  "IO8_FT 100MHz fast speed @ 1.8V"
io8_100m_ft_fs_pu_1v8  "IO8_FT 100MHz fast speed @ 1.8V pullup"
io8_100m_ft_fs_pd_1v8  "IO8_FT 100MHz fast speed @ 1.8V pulldown"
io8_100m_ft_ms_1v8  "IO8_FT 100MHz med speed @ 1.8V"
io8_100m_ft_ms_pu_1v8  "IO8_FT 100MHz med speed @ 1.8V pullup"
io8_100m_ft_ms_pd_1v8  "IO8_FT 100MHz med speed @ 1.8V pulldown"
io8_100m_ft_ls_1v8  "IO8_FT 100MHz low speed @ 1.8V"
io8_100m_ft_ls_pu_1v8  "IO8_FT 100MHz low speed @ 1.8V pullup"
io8_100m_ft_ls_pd_1v8  "IO8_FT 100MHz low speed @ 1.8V pulldown"
io8_100m_ft_hs_3v3  "IO8_FT 100MHz high speed @ 3.3V"
io8_100m_ft_hs_pu_3v3  "IO8_FT 100MHz high speed @ 3.3V pullup"
io8_100m_ft_hs_pd_3v3  "IO8_FT 100MHz high speed @ 3.3V pulldown"
io8_100m_ft_fs_3v3  "IO8_FT 100MHz fast speed @ 3.3V"
io8_100m_ft_fs_pu_3v3  "IO8_FT 100MHz fast speed @ 3.3V pullup"
io8_100m_ft_fs_pd_3v3  "IO8_FT 100MHz fast speed @ 3.3V pulldown"
io8_100m_ft_ms_3v3  "IO8_FT 100MHz med speed @ 3.3V"
io8_100m_ft_ms_pu_3v3  "IO8_FT 100MHz med speed @ 3.3V pullup"
io8_100m_ft_ms_pd_3v3  "IO8_FT 100MHz med speed @ 3.3V pulldown"
io8_100m_ft_ls_3v3  "IO8_FT 100MHz low speed @ 3.3V"
io8_100m_ft_ls_pu_3v3  "IO8_FT 100MHz low speed @ 3.3V pullup"
io8_100m_ft_ls_pd_3v3  "IO8_FT 100MHz low speed @ 3.3V pulldown"
io8usb_adp "IOUSB ADP @ 3.3V"
io8usb_vbus "IOUSB VBUS @ 3.3V"
[Model Selector] io8_166m_hslv_ft
io8_166m_ft_hs_1v2  "IO8_FT 166MHz high speed @ 1.2V"
io8_166m_ft_hs_pu_1v2  "IO8_FT 166MHz high speed @ 1.2V pullup"
io8_166m_ft_hs_pd_1v2  "IO8_FT 166MHz high speed @ 1.2V pulldown"
io8_166m_ft_fs_1v2  "IO8_FT 166MHz fast speed @ 1.2V"
io8_166m_ft_fs_pu_1v2  "IO8_FT 166MHz fast speed @ 1.2V pullup"
io8_166m_ft_fs_pd_1v2  "IO8_FT 166MHz fast speed @ 1.2V pulldown"
io8_166m_ft_ms_1v2  "IO8_FT 166MHz med speed @ 1.2V"
io8_166m_ft_ms_pu_1v2  "IO8_FT 166MHz med speed @ 1.2V pullup"
io8_166m_ft_ms_pd_1v2  "IO8_FT 166MHz med speed @ 1.2V pulldown"
io8_166m_ft_ls_1v2  "IO8_FT 166MHz low speed @ 1.2V"
io8_166m_ft_ls_pu_1v2  "IO8_FT 166MHz low speed @ 1.2V pullup"
io8_166m_ft_ls_pd_1v2  "IO8_FT 166MHz low speed @ 1.2V pulldown"
io8_166m_ft_hs_1v8  "IO8_FT 166MHz high speed @ 1.8V"
io8_166m_ft_hs_pu_1v8  "IO8_FT 166MHz high speed @ 1.8V pullup"
io8_166m_ft_hs_pd_1v8  "IO8_FT 166MHz high speed @ 1.8V pulldown"
io8_166m_ft_fs_1v8  "IO8_FT 166MHz fast speed @ 1.8V"
io8_166m_ft_fs_pu_1v8  "IO8_FT 166MHz fast speed @ 1.8V pullup"
io8_166m_ft_fs_pd_1v8  "IO8_FT 166MHz fast speed @ 1.8V pulldown"
io8_166m_ft_ms_1v8  "IO8_FT 166MHz med speed @ 1.8V"
io8_166m_ft_ms_pu_1v8  "IO8_FT 166MHz med speed @ 1.8V pullup"
io8_166m_ft_ms_pd_1v8  "IO8_FT 166MHz med speed @ 1.8V pulldown"
io8_166m_ft_ls_1v8  "IO8_FT 166MHz low speed @ 1.8V"
io8_166m_ft_ls_pu_1v8  "IO8_FT 166MHz low speed @ 1.8V pullup"
io8_166m_ft_ls_pd_1v8  "IO8_FT 166MHz low speed @ 1.8V pulldown"
io8_166m_ft_hs_3v3  "IO8_FT 166MHz high speed @ 3.3V"
io8_166m_ft_hs_pu_3v3  "IO8_FT 166MHz high speed @ 3.3V pullup"
io8_166m_ft_hs_pd_3v3  "IO8_FT 166MHz high speed @ 3.3V pulldown"
io8_166m_ft_fs_3v3  "IO8_FT 166MHz fast speed @ 3.3V"
io8_166m_ft_fs_pu_3v3  "IO8_FT 166MHz fast speed @ 3.3V pullup"
io8_166m_ft_fs_pd_3v3  "IO8_FT 166MHz fast speed @ 3.3V pulldown"
io8_166m_ft_ms_3v3  "IO8_FT 166MHz med speed @ 3.3V"
io8_166m_ft_ms_pu_3v3  "IO8_FT 166MHz med speed @ 3.3V pullup"
io8_166m_ft_ms_pd_3v3  "IO8_FT 166MHz med speed @ 3.3V pulldown"
io8_166m_ft_ls_3v3  "IO8_FT 166MHz low speed @ 3.3V"
io8_166m_ft_ls_pu_3v3  "IO8_FT 166MHz low speed @ 3.3V pullup"
io8_166m_ft_ls_pd_3v3  "IO8_FT 166MHz low speed @ 3.3V pulldown"
io8_166m_hslv_ft_hs_1v2  "IO8_FT 166MHz HSLV high speed @ 1.2V"
io8_166m_hslv_ft_hs_pu_1v2  "IO8_FT 166MHz HSLV high speed @ 1.2V pullup"
io8_166m_hslv_ft_hs_pd_1v2  "IO8_FT 166MHz HSLV high speed @ 1.2V pulldown"
io8_166m_hslv_ft_fs_1v2  "IO8_FT 166MHz HSLV fast speed @ 1.2V"
io8_166m_hslv_ft_fs_pu_1v2  "IO8_FT 166MHz HSLV fast speed @ 1.2V pullup"
io8_166m_hslv_ft_fs_pd_1v2  "IO8_FT 166MHz HSLV fast speed @ 1.2V pulldown"
io8_166m_hslv_ft_ms_1v2  "IO8_FT 166MHz HSLV med speed @ 1.2V"
io8_166m_hslv_ft_ms_pu_1v2  "IO8_FT 166MHz HSLV med speed @ 1.2V pullup"
io8_166m_hslv_ft_ms_pd_1v2  "IO8_FT 166MHz HSLV med speed @ 1.2V pulldown"
io8_166m_hslv_ft_ls_1v2  "IO8_FT 166MHz HSLV low speed @ 1.2V"
io8_166m_hslv_ft_ls_pu_1v2  "IO8_FT 166MHz HSLV low speed @ 1.2V pullup"
io8_166m_hslv_ft_ls_pd_1v2  "IO8_FT 166MHz HSLV low speed @ 1.2V pulldown"
io8_166m_hslv_ft_hs_1v8  "IO8_FT 166MHz HSLV high speed @ 1.8V"
io8_166m_hslv_ft_hs_pu_1v8  "IO8_FT 166MHz HSLV high speed @ 1.8V pullup"
io8_166m_hslv_ft_hs_pd_1v8  "IO8_FT 166MHz HSLV high speed @ 1.8V pulldown"
io8_166m_hslv_ft_fs_1v8  "IO8_FT 166MHz HSLV fast speed @ 1.8V"
io8_166m_hslv_ft_fs_pu_1v8  "IO8_FT 166MHz HSLV fast speed @ 1.8V pullup"
io8_166m_hslv_ft_fs_pd_1v8  "IO8_FT 166MHz HSLV fast speed @ 1.8V pulldown"
io8_166m_hslv_ft_ms_1v8  "IO8_FT 166MHz HSLV med speed @ 1.8V"
io8_166m_hslv_ft_ms_pu_1v8  "IO8_FT 166MHz HSLV med speed @ 1.8V pullup"
io8_166m_hslv_ft_ms_pd_1v8  "IO8_FT 166MHz HSLV med speed @ 1.8V pulldown"
io8_166m_hslv_ft_ls_1v8  "IO8_FT 166MHz HSLV low speed @ 1.8V"
io8_166m_hslv_ft_ls_pu_1v8  "IO8_FT 166MHz HSLV low speed @ 1.8V pullup"
io8_166m_hslv_ft_ls_pd_1v8  "IO8_FT 166MHz HSLV low speed @ 1.8V pulldown"
io8_166m_hslv_ft_hs_2v5  "IO8_FT 166MHz HSLV high speed @ 2.5V"
io8_166m_hslv_ft_hs_pu_2v5  "IO8_FT 166MHz HSLV high speed @ 2.5V pullup"
io8_166m_hslv_ft_hs_pd_2v5  "IO8_FT 166MHz HSLV high speed @ 2.5V pulldown"
io8_166m_hslv_ft_fs_2v5  "IO8_FT 166MHz HSLV fast speed @ 2.5V"
io8_166m_hslv_ft_fs_pu_2v5  "IO8_FT 166MHz HSLV fast speed @ 2.5V pullup"
io8_166m_hslv_ft_fs_pd_2v5  "IO8_FT 166MHz HSLV fast speed @ 2.5V pulldown"
io8_166m_hslv_ft_ms_2v5  "IO8_FT 166MHz HSLV med speed @ 2.5V"
io8_166m_hslv_ft_ms_pu_2v5  "IO8_FT 166MHz HSLV med speed @ 2.5V pullup"
io8_166m_hslv_ft_ms_pd_2v5  "IO8_FT 166MHz HSLV med speed @ 2.5V pulldown"
io8_166m_hslv_ft_ls_2v5  "IO8_FT 166MHz HSLV low speed @ 2.5V"
io8_166m_hslv_ft_ls_pu_2v5  "IO8_FT 166MHz HSLV low speed @ 2.5V pullup"
io8_166m_hslv_ft_ls_pd_2v5  "IO8_FT 166MHz HSLV low speed @ 2.5V pulldown"
[Model Selector] io8_spi_hslv_ft
io8_spi_ft_hs_1v2  "IO8_FT SPI high speed @ 1.2V"
io8_spi_ft_hs_pu_1v2  "IO8_FT SPI high speed @ 1.2V pullup"
io8_spi_ft_hs_pd_1v2  "IO8_FT SPI high speed @ 1.2V pulldown"
io8_spi_ft_fs_1v2  "IO8_FT SPI fast speed @ 1.2V"
io8_spi_ft_fs_pu_1v2  "IO8_FT SPI fast speed @ 1.2V pullup"
io8_spi_ft_fs_pd_1v2  "IO8_FT SPI fast speed @ 1.2V pulldown"
io8_spi_ft_ms_1v2  "IO8_FT SPI med speed @ 1.2V"
io8_spi_ft_ms_pu_1v2  "IO8_FT SPI med speed @ 1.2V pullup"
io8_spi_ft_ms_pd_1v2  "IO8_FT SPI med speed @ 1.2V pulldown"
io8_spi_ft_ls_1v2  "IO8_FT SPI low speed @ 1.2V"
io8_spi_ft_ls_pu_1v2  "IO8_FT SPI low speed @ 1.2V pullup"
io8_spi_ft_ls_pd_1v2  "IO8_FT SPI low speed @ 1.2V pulldown"
io8_spi_ft_hs_1v8  "IO8_FT SPI high speed @ 1.8V"
io8_spi_ft_hs_pu_1v8  "IO8_FT SPI high speed @ 1.8V pullup"
io8_spi_ft_hs_pd_1v8  "IO8_FT SPI high speed @ 1.8V pulldown"
io8_spi_ft_fs_1v8  "IO8_FT SPI fast speed @ 1.8V"
io8_spi_ft_fs_pu_1v8  "IO8_FT SPI fast speed @ 1.8V pullup"
io8_spi_ft_fs_pd_1v8  "IO8_FT SPI fast speed @ 1.8V pulldown"
io8_spi_ft_ms_1v8  "IO8_FT SPI med speed @ 1.8V"
io8_spi_ft_ms_pu_1v8  "IO8_FT SPI med speed @ 1.8V pullup"
io8_spi_ft_ms_pd_1v8  "IO8_FT SPI med speed @ 1.8V pulldown"
io8_spi_ft_ls_1v8  "IO8_FT SPI low speed @ 1.8V"
io8_spi_ft_ls_pu_1v8  "IO8_FT SPI low speed @ 1.8V pullup"
io8_spi_ft_ls_pd_1v8  "IO8_FT SPI low speed @ 1.8V pulldown"
io8_spi_ft_hs_3v3  "IO8_FT SPI high speed @ 3.3V"
io8_spi_ft_hs_pu_3v3  "IO8_FT SPI high speed @ 3.3V pullup"
io8_spi_ft_hs_pd_3v3  "IO8_FT SPI high speed @ 3.3V pulldown"
io8_spi_ft_fs_3v3  "IO8_FT SPI fast speed @ 3.3V"
io8_spi_ft_fs_pu_3v3  "IO8_FT SPI fast speed @ 3.3V pullup"
io8_spi_ft_fs_pd_3v3  "IO8_FT SPI fast speed @ 3.3V pulldown"
io8_spi_ft_ms_3v3  "IO8_FT SPI med speed @ 3.3V"
io8_spi_ft_ms_pu_3v3  "IO8_FT SPI med speed @ 1.8V pullup"
io8_spi_ft_ms_pd_3v3  "IO8_FT SPI med speed @ 3.3V pulldown"
io8_spi_ft_ls_3v3  "IO8_FT SPI low speed @ 3.3V"
io8_spi_ft_ls_pu_3v3  "IO8_FT SPI low speed @ 3.3V pullup"
io8_spi_ft_ls_pd_3v3  "IO8_FT SPI low speed @ 3.3V pulldown"
io8_spi_hslv_ft_hs_1v2  "IO8_FT SPI HSLV high speed @ 1.2V"
io8_spi_hslv_ft_hs_pu_1v2  "IO8_FT SPI HSLV high speed @ 1.2V pullup"
io8_spi_hslv_ft_hs_pd_1v2  "IO8_FT SPI HSLV high speed @ 1.2V pulldown"
io8_spi_hslv_ft_fs_1v2  "IO8_FT SPI HSLV fast speed @ 1.2V"
io8_spi_hslv_ft_fs_pu_1v2  "IO8_FT SPI HSLV fast speed @ 1.2V pullup"
io8_spi_hslv_ft_fs_pd_1v2  "IO8_FT SPI HSLV fast speed @ 1.2V pulldown"
io8_spi_hslv_ft_ms_1v2  "IO8_FT SPI HSLV med speed @ 1.2V"
io8_spi_hslv_ft_ms_pu_1v2  "IO8_FT SPI HSLV med speed @ 1.2V pullup"
io8_spi_hslv_ft_ms_pd_1v2  "IO8_FT SPI HSLV med speed @ 1.2V pulldown"
io8_spi_hslv_ft_ls_1v2  "IO8_FT SPI HSLV low speed @ 1.2V"
io8_spi_hslv_ft_ls_pu_1v2  "IO8_FT SPI HSLV low speed @ 1.2V pullup"
io8_spi_hslv_ft_ls_pd_1v2  "IO8_FT SPI HSLV low speed @ 1.2V pulldown"
io8_spi_hslv_ft_hs_1v8  "IO8_FT SPI HSLV high speed @ 1.8V"
io8_spi_hslv_ft_hs_pu_1v8  "IO8_FT SPI HSLV high speed @ 1.8V pullup"
io8_spi_hslv_ft_hs_pd_1v8  "IO8_FT SPI HSLV high speed @ 1.8V pulldown"
io8_spi_hslv_ft_fs_1v8  "IO8_FT SPI HSLV fast speed @ 1.8V"
io8_spi_hslv_ft_fs_pu_1v8  "IO8_FT SPI HSLV fast speed @ 1.8V pullup"
io8_spi_hslv_ft_fs_pd_1v8  "IO8_FT SPI HSLV fast speed @ 1.8V pulldown"
io8_spi_hslv_ft_ms_1v8  "IO8_FT SPI HSLV med speed @ 1.8V"
io8_spi_hslv_ft_ms_pu_1v8  "IO8_FT SPI HSLV med speed @ 1.8V pullup"
io8_spi_hslv_ft_ms_pd_1v8  "IO8_FT SPI HSLV med speed @ 1.8V pulldown"
io8_spi_hslv_ft_ls_1v8  "IO8_FT SPI HSLV low speed @ 1.8V"
io8_spi_hslv_ft_ls_pu_1v8  "IO8_FT SPI HSLV low speed @ 1.8V pullup"
io8_spi_hslv_ft_ls_pd_1v8  "IO8_FT SPI HSLV low speed @ 1.8V pulldown"
io8_spi_hslv_ft_hs_2v5  "IO8_FT SPI HSLV high speed @ 2.5V"
io8_spi_hslv_ft_hs_pu_2v5  "IO8_FT SPI HSLV high speed @ 2.5V pullup"
io8_spi_hslv_ft_hs_pd_2v5  "IO8_FT SPI HSLV high speed @ 2.5V pulldown"
io8_spi_hslv_ft_fs_2v5  "IO8_FT SPI HSLV fast speed @ 2.5V"
io8_spi_hslv_ft_fs_pu_2v5  "IO8_FT SPI HSLV fast speed @ 2.5V pullup"
io8_spi_hslv_ft_fs_pd_2v5  "IO8_FT SPI HSLV fast speed @ 2.5V pulldown"
io8_spi_hslv_ft_ms_2v5  "IO8_FT SPI HSLV med speed @ 2.5V"
io8_spi_hslv_ft_ms_pu_2v5  "IO8_FT SPI HSLV med speed @ 2.5V pullup"
io8_spi_hslv_ft_ms_pd_2v5  "IO8_FT SPI HSLV med speed @ 2.5V pulldown"
io8_spi_hslv_ft_ls_2v5  "IO8_FT SPI HSLV low speed @ 2.5V"
io8_spi_hslv_ft_ls_pu_2v5  "IO8_FT SPI HSLV low speed @ 2.5V pullup"
io8_spi_hslv_ft_ls_pd_2v5  "IO8_FT SPI HSLV low speed @ 2.5V pulldown"
[Model Selector] io8_spi_ft
io8_spi_ft_hs_1v2  "IO8_FT SPI high speed @ 1.2V"
io8_spi_ft_hs_pu_1v2  "IO8_FT SPI high speed @ 1.2V pullup"
io8_spi_ft_hs_pd_1v2  "IO8_FT SPI high speed @ 1.2V pulldown"
io8_spi_ft_fs_1v2  "IO8_FT SPI fast speed @ 1.2V"
io8_spi_ft_fs_pu_1v2  "IO8_FT SPI fast speed @ 1.2V pullup"
io8_spi_ft_fs_pd_1v2  "IO8_FT SPI fast speed @ 1.2V pulldown"
io8_spi_ft_ms_1v2  "IO8_FT SPI med speed @ 1.2V"
io8_spi_ft_ms_pu_1v2  "IO8_FT SPI med speed @ 1.2V pullup"
io8_spi_ft_ms_pd_1v2  "IO8_FT SPI med speed @ 1.2V pulldown"
io8_spi_ft_ls_1v2  "IO8_FT SPI low speed @ 1.2V"
io8_spi_ft_ls_pu_1v2  "IO8_FT SPI low speed @ 1.2V pullup"
io8_spi_ft_ls_pd_1v2  "IO8_FT SPI low speed @ 1.2V pulldown"
io8_spi_ft_hs_1v8  "IO8_FT SPI high speed @ 1.8V"
io8_spi_ft_hs_pu_1v8  "IO8_FT SPI high speed @ 1.8V pullup"
io8_spi_ft_hs_pd_1v8  "IO8_FT SPI high speed @ 1.8V pulldown"
io8_spi_ft_fs_1v8  "IO8_FT SPI fast speed @ 1.8V"
io8_spi_ft_fs_pu_1v8  "IO8_FT SPI fast speed @ 1.8V pullup"
io8_spi_ft_fs_pd_1v8  "IO8_FT SPI fast speed @ 1.8V pulldown"
io8_spi_ft_ms_1v8  "IO8_FT SPI med speed @ 1.8V"
io8_spi_ft_ms_pu_1v8  "IO8_FT SPI med speed @ 1.8V pullup"
io8_spi_ft_ms_pd_1v8  "IO8_FT SPI med speed @ 1.8V pulldown"
io8_spi_ft_ls_1v8  "IO8_FT SPI low speed @ 1.8V"
io8_spi_ft_ls_pu_1v8  "IO8_FT SPI low speed @ 1.8V pullup"
io8_spi_ft_ls_pd_1v8  "IO8_FT SPI low speed @ 1.8V pulldown"
io8_spi_ft_hs_3v3  "IO8_FT SPI high speed @ 3.3V"
io8_spi_ft_hs_pu_3v3  "IO8_FT SPI high speed @ 3.3V pullup"
io8_spi_ft_hs_pd_3v3  "IO8_FT SPI high speed @ 3.3V pulldown"
io8_spi_ft_fs_3v3  "IO8_FT SPI fast speed @ 3.3V"
io8_spi_ft_fs_pu_3v3  "IO8_FT SPI fast speed @ 3.3V pullup"
io8_spi_ft_fs_pd_3v3  "IO8_FT SPI fast speed @ 3.3V pulldown"
io8_spi_ft_ms_3v3  "IO8_FT SPI med speed @ 3.3V"
io8_spi_ft_ms_pu_3v3  "IO8_FT SPI med speed @ 1.8V pullup"
io8_spi_ft_ms_pd_3v3  "IO8_FT SPI med speed @ 3.3V pulldown"
io8_spi_ft_ls_3v3  "IO8_FT SPI low speed @ 3.3V"
io8_spi_ft_ls_pu_3v3  "IO8_FT SPI low speed @ 3.3V pullup"
io8_spi_ft_ls_pd_3v3  "IO8_FT SPI low speed @ 3.3V pulldown"
io8_spi_hslv_ft_hs_1v2  "IO8_FT SPI HSLV high speed @ 1.2V"
io8_spi_hslv_ft_hs_pu_1v2  "IO8_FT SPI HSLV high speed @ 1.2V pullup"
io8_spi_hslv_ft_hs_pd_1v2  "IO8_FT SPI HSLV high speed @ 1.2V pulldown"
io8_spi_hslv_ft_fs_1v2  "IO8_FT SPI HSLV fast speed @ 1.2V"
io8_spi_hslv_ft_fs_pu_1v2  "IO8_FT SPI HSLV fast speed @ 1.2V pullup"
io8_spi_hslv_ft_fs_pd_1v2  "IO8_FT SPI HSLV fast speed @ 1.2V pulldown"
io8_spi_hslv_ft_ms_1v2  "IO8_FT SPI HSLV med speed @ 1.2V"
io8_spi_hslv_ft_ms_pu_1v2  "IO8_FT SPI HSLV med speed @ 1.2V pullup"
io8_spi_hslv_ft_ms_pd_1v2  "IO8_FT SPI HSLV med speed @ 1.2V pulldown"
io8_spi_hslv_ft_ls_1v2  "IO8_FT SPI HSLV low speed @ 1.2V"
io8_spi_hslv_ft_ls_pu_1v2  "IO8_FT SPI HSLV low speed @ 1.2V pullup"
io8_spi_hslv_ft_ls_pd_1v2  "IO8_FT SPI HSLV low speed @ 1.2V pulldown"
io8_spi_hslv_ft_hs_1v8  "IO8_FT SPI HSLV high speed @ 1.8V"
io8_spi_hslv_ft_hs_pu_1v8  "IO8_FT SPI HSLV high speed @ 1.8V pullup"
io8_spi_hslv_ft_hs_pd_1v8  "IO8_FT SPI HSLV high speed @ 1.8V pulldown"
io8_spi_hslv_ft_fs_1v8  "IO8_FT SPI HSLV fast speed @ 1.8V"
io8_spi_hslv_ft_fs_pu_1v8  "IO8_FT SPI HSLV fast speed @ 1.8V pullup"
io8_spi_hslv_ft_fs_pd_1v8  "IO8_FT SPI HSLV fast speed @ 1.8V pulldown"
io8_spi_hslv_ft_ms_1v8  "IO8_FT SPI HSLV med speed @ 1.8V"
io8_spi_hslv_ft_ms_pu_1v8  "IO8_FT SPI HSLV med speed @ 1.8V pullup"
io8_spi_hslv_ft_ms_pd_1v8  "IO8_FT SPI HSLV med speed @ 1.8V pulldown"
io8_spi_hslv_ft_ls_1v8  "IO8_FT SPI HSLV low speed @ 1.8V"
io8_spi_hslv_ft_ls_pu_1v8  "IO8_FT SPI HSLV low speed @ 1.8V pullup"
io8_spi_hslv_ft_ls_pd_1v8  "IO8_FT SPI HSLV low speed @ 1.8V pulldown"
io8_spi_hslv_ft_hs_2v5  "IO8_FT SPI HSLV high speed @ 2.5V"
io8_spi_hslv_ft_hs_pu_2v5  "IO8_FT SPI HSLV high speed @ 2.5V pullup"
io8_spi_hslv_ft_hs_pd_2v5  "IO8_FT SPI HSLV high speed @ 2.5V pulldown"
io8_spi_hslv_ft_fs_2v5  "IO8_FT SPI HSLV fast speed @ 2.5V"
io8_spi_hslv_ft_fs_pu_2v5  "IO8_FT SPI HSLV fast speed @ 2.5V pullup"
io8_spi_hslv_ft_fs_pd_2v5  "IO8_FT SPI HSLV fast speed @ 2.5V pulldown"
io8_spi_hslv_ft_ms_2v5  "IO8_FT SPI HSLV med speed @ 2.5V"
io8_spi_hslv_ft_ms_pu_2v5  "IO8_FT SPI HSLV med speed @ 2.5V pullup"
io8_spi_hslv_ft_ms_pd_2v5  "IO8_FT SPI HSLV med speed @ 2.5V pulldown"
io8_spi_hslv_ft_ls_2v5  "IO8_FT SPI HSLV low speed @ 2.5V"
io8_spi_hslv_ft_ls_pu_2v5  "IO8_FT SPI HSLV low speed @ 2.5V pullup"
io8_spi_hslv_ft_ls_pd_2v5  "IO8_FT SPI HSLV low speed @ 2.5V pulldown"
[Define Package Model]  481-tfbga-13x13-216-220909
[Manufacturer]  unknown
[OEM]  unknown
[Description]  unknown
[Number Of Pins]  186
[Pin Numbers]
| Pin Name Terminal   Net Name   Starting Node   Ending Node
J1 | DSI_CKN
H1 | DSI_CKP
G2 | DSI_D0N
G1 | DSI_D0P
K1 | DSI_D1N
K2 | DSI_D1P
R2 | NRST
R3 | OPAMP1_VINM
N5 | OPAMP2_VINM
N4 | PA0
P3 | PA1
M4 | PA2
P4 | PA3
M5 | PA4
R4 | PA5
P5 | PA6
R5 | PA7
A13 | PA8
E12 | PA9
D12 | PA10
B14 | PA11
B13 | PA12
C13 | PA13
A12 | PA14
A11 | PA15
N6 | PB0
M6 | PB1
R7 | PB2
E7 | PB3
D6 | PB4
B5 | PB5
A4 | PB6
A3 | PB7
C6 | PB8
C5 | PB9
N12 | PB10
M10 | PB11
M11 | PB12
M12 | PB13
P13 | PB14
R14 | PB15
P2 | PC0
M1 | PC1
P1 | PC2
N3 | PC3
R6 | PC4
P6 | PC5
C15 | PC6
B15 | PC7
A14 | PC8
C14 | PC9
A10 | PC10
B10 | PC11
C10 | PC12
F4 | PC13
B1 | PC14-OSC32_IN
C1 | PC15-OSC32_OUT
D9 | PD0
C9 | PD1
B9 | PD2
A9 | PD3
A8 | PD4
B8 | PD5
C8 | PD6
D8 | PD7
N13 | PD8
P15 | PD9
P14 | PD10
L12 | PD11
M13 | PD12
N14 | PD13
N15 | PD14
K12 | PD15
A2 | PE0
B3 | PE1
E5 | PE2
C3 | PE3
B2 | PE4
D3 | PE5
E4 | PE6
N9 | PE7
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| Models and submodels in the file (265): io8_100m_ft_hs_1v2 (I/O), io8_100m_ft_hs_pu_1v2 (I/O), io8_100m_ft_hs_pd_1v2 (I/O), io8_100m_ft_fs_1v2 (I/O), io8_100m_ft_fs_pu_1v2 (I/O), io8_100m_ft_fs_pd_1v2 (I/O), io8_100m_ft_ms_1v2 (I/O), io8_100m_ft_ms_pu_1v2 (I/O), io8_100m_ft_ms_pd_1v2 (I/O), io8_100m_ft_ls_1v2 (I/O), io8_100m_ft_ls_pu_1v2 (I/O), io8_100m_ft_ls_pd_1v2 (I/O), io8_100m_ft_hs_1v8 (I/O), io8_100m_ft_hs_pu_1v8 (I/O), io8_100m_ft_hs_pd_1v8 (I/O), io8_100m_ft_fs_1v8 (I/O), io8_100m_ft_fs_pu_1v8 (I/O), io8_100m_ft_fs_pd_1v8 (I/O), io8_100m_ft_ms_1v8 (I/O), io8_100m_ft_ms_pu_1v8 (I/O), io8_100m_ft_ms_pd_1v8 (I/O), io8_100m_ft_ls_1v8 (I/O), io8_100m_ft_ls_pu_1v8 (I/O), io8_100m_ft_ls_pd_1v8 (I/O), io8_100m_ft_hs_3v3 (I/O), io8_100m_ft_hs_pu_3v3 (I/O), io8_100m_ft_hs_pd_3v3 (I/O), io8_100m_ft_fs_3v3 (I/O), io8_100m_ft_fs_pu_3v3 (I/O), io8_100m_ft_fs_pd_3v3 (I/O), io8_100m_ft_ms_3v3 (I/O), io8_100m_ft_ms_pu_3v3 (I/O), io8_100m_ft_ms_pd_3v3 (I/O), io8_100m_ft_ls_3v3 (I/O), io8_100m_ft_ls_pu_3v3 (I/O), io8_100m_ft_ls_pd_3v3 (I/O), io8_100m_hslv_ft_hs_1v2 (I/O), io8_100m_hslv_ft_hs_pu_1v2 (I/O), io8_100m_hslv_ft_hs_pd_1v2 (I/O), io8_100m_hslv_ft_fs_1v2 (I/O), io8_100m_hslv_ft_fs_pu_1v2 (I/O), io8_100m_hslv_ft_fs_pd_1v2 (I/O), io8_100m_hslv_ft_ms_1v2 (I/O), io8_100m_hslv_ft_ms_pu_1v2 (I/O), io8_100m_hslv_ft_ms_pd_1v2 (I/O), io8_100m_hslv_ft_ls_1v2 (I/O), io8_100m_hslv_ft_ls_pu_1v2 (I/O), io8_100m_hslv_ft_ls_pd_1v2 (I/O), io8_100m_hslv_ft_hs_1v8 (I/O), io8_100m_hslv_ft_hs_pu_1v8 (I/O), io8_100m_hslv_ft_hs_pd_1v8 (I/O), io8_100m_hslv_ft_fs_1v8 (I/O), io8_100m_hslv_ft_fs_pu_1v8 (I/O), io8_100m_hslv_ft_fs_pd_1v8 (I/O), io8_100m_hslv_ft_ms_1v8 (I/O), io8_100m_hslv_ft_ms_pu_1v8 (I/O), io8_100m_hslv_ft_ms_pd_1v8 (I/O), io8_100m_hslv_ft_ls_1v8 (I/O), io8_100m_hslv_ft_ls_pu_1v8 (I/O), io8_100m_hslv_ft_ls_pd_1v8 (I/O), io8_100m_hslv_ft_hs_2v5 (I/O), io8_100m_hslv_ft_hs_pu_2v5 (I/O), io8_100m_hslv_ft_hs_pd_2v5 (I/O), io8_100m_hslv_ft_fs_2v5 (I/O), io8_100m_hslv_ft_fs_pu_2v5 (I/O), io8_100m_hslv_ft_fs_pd_2v5 (I/O), io8_100m_hslv_ft_ms_2v5 (I/O), io8_100m_hslv_ft_ms_pu_2v5 (I/O), io8_100m_hslv_ft_ms_pd_2v5 (I/O), io8_100m_hslv_ft_ls_2v5 (I/O), io8_100m_hslv_ft_ls_pu_2v5 (I/O), io8_100m_hslv_ft_ls_pd_2v5 (I/O), io8_100m_i2c_ft_1v2 (I/O_open_drain), io8_100m_i2c_ft_pu_1v2 (I/O_open_drain), io8_100m_i2c_ft_pd_1v2 (I/O_open_drain), io8_100m_i2c_ft_1v8 (I/O_open_drain), io8_100m_i2c_ft_pu_1v8 (I/O_open_drain), io8_100m_i2c_ft_pd_1v8 (I/O_open_drain), io8_100m_i2c_ft_3v3 (I/O_open_drain), io8_100m_i2c_ft_pu_3v3 (I/O_open_drain)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
